PROGRAM MAIN
VAR
	IC_KP2_2HB21_IUH_MF_Head1	: IC_KP2_2HB21_IUH_MF;		(*Function block for channel 1 to read/write data and parameter access for IUH-F19x-V1-FRx-xx MultiFrame Protocol*)
	IC_KP2_2HB21_IUH_MF_Head2	: IC_KP2_2HB21_IUH_MF;		(*Function block for channel 2 to read/write data and parameter access for IUH-F19x-V1-FRx-xx MultiFrame Protocol*)
	
	Head1Data					: IDENTControl_UserData_IUH_MF;	(*Data block for read/write data and parameter data of channel 1*)
	Head2Data 					: IDENTControl_UserData_IUH_MF;	(*Data block for read/write data and parameter data of channel 2*)
		
	Head1SetRestart				: BOOL;						(*Trigger initialisation routine*)
	Head1InitFinish				: BOOL;						(*Initialisation routine finished*)
	Head1Quit					: BOOL;						(*Trigger Quit command to about Enhanced command*)
	Head1Read					: BOOL;						(*Trigger Read command*)
	Head1UserMemoryUID			: BOOL;						(*0 := access to User Memory; 1 := access to TID/Fixcode*)		
	Head1EPC 					: BOOL;						(*0 := configuration done by Head1UserMemoryUID active; 1 := access to UII/EPC Code (UHF only)*)
	Head1Busy					: BOOL;						(*0 = no command actiive; 1 = command active*)
	Head1Done					: BOOL;						(*0 = tag leave detection zone (Enhanced); 1 = tag access successfully executed*)
	Head1Finish 				: BOOL;						(*0 = command active; 1 = command finished*)		
	Head1Status					: BYTE;						(*Status value of the command response; error information*)
	Head1ReplyCounter			: BYTE;						(*Counter of the command responses; increment each new response*)
	Head1Error					: BOOL;						(*0 = no error state; 1 = error state active; check status value*)
	Head1SingleEnhanced			: BOOL;						(*0 := execute a Single (one-time) command; 1 := execute an Enhanced (permanent) command*)
	Head1NoDataCarrier			: BOOL;						(*0 = tag inside/enter detection zone; 1 = no tag or tag leave detection zone*)
	Head1Write					: BOOL;						(*Trigger Write command*)
	Head1TagType 				: WORD := 16#3830;			(*Configuration of TagType; default = 16#3939 = "99"; for IUH-F19x-V1-FRx-xx use 16#3830*)
	Head1StartAddress 			: WORD := 16#0000;			(*Configuration of start address on User Memory for tag access*)
	Head1WordNum 				: INT := 4;					(*Number of accessed 2-Byte words*)
	Head1SpecialCommand			: BOOL;						(*Trigger Special (user defined) command*)
	Head1StartConfig			: BOOL;						(*Trigger to start parameter access*)
	Head1EndConfig 				: BOOL;						(*1 = parameter access finished*)
	Head1WriteParameter			: BOOL;						(*0 = read parameter; 1 = write parameter*)
	Head1NewData				: BOOL;						(*1 = new data inside data block aviable; direct reset by the user neccessary*)
	
	Head2SetRestart				: BOOL;						(*Trigger initialisation routine*)
	Head2InitFinish				: BOOL;						(*Initialisation routine finished*)
	Head2Quit					: BOOL;						(*Trigger Quit command to about Enhanced command*)
	Head2Read					: BOOL;						(*Trigger Read command*)
	Head2UserMemoryUID			: BOOL;						(*0 := access to User Memory; 1 := access to TID/Fixcode*)
	Head2EPC 					: BOOL;						(*0 := configuration done by Head2UserMemoryUID active; 1 := access to UII/EPC Code (UHF only)*)
	Head2Busy					: BOOL;						(*0 = no command actiive; 1 = command active*)
	Head2Done					: BOOL;						(*0 = tag leave detection zone (Enhanced); 1 = tag access successfully executed*)
	Head2Finish 				: BOOL;						(*0 = command active; 1 = command finished*)	
	Head2Status					: BYTE;						(*Status value of the command response; error information*)
	Head2ReplyCounter			: BYTE;						(*Counter of the command responses; increment each new response*)
	Head2Error					: BOOL;						(*0 = no error state; 1 = error state active; check status value*)
	Head2SingleEnhanced			: BOOL;						(*0 := execute a Single (one-time) command; 1 := execute an Enhanced (permanent) command*)
	Head2NoDataCarrier			: BOOL;						(*0 = tag inside/enter detection zone; 1 = no tag or tag leave detection zone*)
	Head2Write					: BOOL;						(*Trigger Write command*)
	Head2TagType 				: WORD := 16#3830;			(*Configuration of TagType; default = 16#3939 = "99"; for IUH-F19x-V1-FRx-xx use 16#3830*)
	Head2StartAddress 			: WORD := 16#0000;			(*Configuration of start address on User Memory for tag access*)
	Head2WordNum 				: INT := 4;					(*Number of accessed 2-Byte words*)
	Head2SpecialCommand			: BOOL;						(*Trigger Special (user defined) command*)
	Head2StartConfig			: BOOL;						(*Trigger to start parameter access*)
	Head2EndConfig 				: BOOL;						(*1 = parameter access finished*)
	Head2WriteParameter			: BOOL;						(*0 = read parameter; 1 = write parameter*)
	Head2NewData				: BOOL;						(*1 = new data inside data block aviable; direct reset by the user neccessary*)
END_VAR


//Call function block for channel 1
IC_KP2_2HB21_IUH_MF_Head1(
	pADR_IN	:= ADR(BUS_INPUT[1]),						(* Pointer array input data *)
	cbSIZE_IN := SIZEOF(BUS_INPUT[1]),					(* Size array input data *)
	pADR_OUT := ADR(BUS_OUTPUT[1]),						(* Pointer array output data *)
	cbSIZE_OUT := SIZEOF(BUS_OUTPUT[1]), 
	I_T_Timeout := T#5S,
	I_b_StartRead:= Head1Read, 
	I_b_StartWrite:= Head1Write, 
	I_b_StartSpecialCommand:= Head1Specialcommand, 
	I_b_UserMemory_UID:= Head1UserMemoryUID, 
	I_b_EPC:= Head1EPC, 
	I_b_SingleEnhanced:= Head1SingleEnhanced, 
	I_b_Quit:= Head1Quit, 
	I_w_StartAddress:= Head1Startaddress, 
	I_i_WordNumber:= Head1WordNum, 
	I_w_TagType:= 16#3830, 
	I_b_WriteParameter := Head1WriteParameter,
	O_b_Done=> Head1Done , 
	O_b_NoDataCarrier=> Head1NoDataCarrier, 
	O_b_Busy=> Head1Busy, 
	O_b_Finish=> Head1Finish, 
	O_b_Error=> Head1Error, 
	O_B_Status=> Head1Status, 
	O_B_ReplyCounter=> Head1ReplyCounter , 
	O_b_EndConfig => Head1EndConfig,
	IO_b_SetRestart:= Head1SetRestart, 
	IO_b_InitFinish:= Head1InitFinish,
	IO_b_StartConfig := Head1StartConfig, 
	IO_b_NewData := Head1NewData,
	UserDataGlobal:= Head1Data);	

IF Head1Read = TRUE THEN Head1Read := FALSE; END_IF;
IF Head1Write = TRUE THEN Head1Write := FALSE; END_IF;
IF Head1Quit = TRUE THEN Head1Quit := FALSE; END_IF;
IF Head1SpecialCommand = TRUE THEN Head1SpecialCommand := FALSE; END_IF;


//Call function block for channel 2
IC_KP2_2HB21_IUH_MF_Head2(
	pADR_IN	:= ADR(BUS_INPUT[2]),						(* Pointer array input data *)
	cbSIZE_IN := SIZEOF(BUS_INPUT[2]),					(* Size array input data *)
	pADR_OUT := ADR(BUS_OUTPUT[2]),						(* Pointer array output data *)
	cbSIZE_OUT := SIZEOF(BUS_OUTPUT[2]), 
	I_T_Timeout := T#5S,
	I_b_StartRead:= Head2Read, 
	I_b_StartWrite:= Head2Write, 
	I_b_StartSpecialCommand:= Head2Specialcommand, 
	I_b_UserMemory_UID:= Head2UserMemoryUID, 
	I_b_EPC:= Head2EPC, 
	I_b_SingleEnhanced:= Head2SingleEnhanced, 
	I_b_Quit:= Head2Quit, 
	I_w_StartAddress:= Head2Startaddress, 
	I_i_WordNumber:= Head2WordNum, 
	I_w_TagType:= Head2TagType, 
	I_b_WriteParameter := Head2WriteParameter,
	O_b_Done=> Head2Done , 
	O_b_NoDataCarrier=> Head2NoDataCarrier, 
	O_b_Busy=> Head2Busy, 
	O_b_Finish=> Head2Finish, 
	O_b_Error=> Head2Error, 
	O_B_Status=> Head2Status, 
	O_B_ReplyCounter=> Head2ReplyCounter , 
	O_b_EndConfig => Head2EndConfig,
	IO_b_SetRestart:= Head2SetRestart, 
	IO_b_InitFinish:= Head2InitFinish,
	IO_b_StartConfig := Head2StartConfig, 
	IO_b_NewData := Head2NewData,
	UserDataGlobal:= Head2Data);	

IF Head2Read = TRUE THEN Head2Read := FALSE; END_IF;
IF Head2Write = TRUE THEN Head2Write := FALSE; END_IF;
IF Head2Quit = TRUE THEN Head2Quit := FALSE; END_IF;
IF Head2SpecialCommand = TRUE THEN Head2SpecialCommand := FALSE; END_IF;

END_PROGRAM
